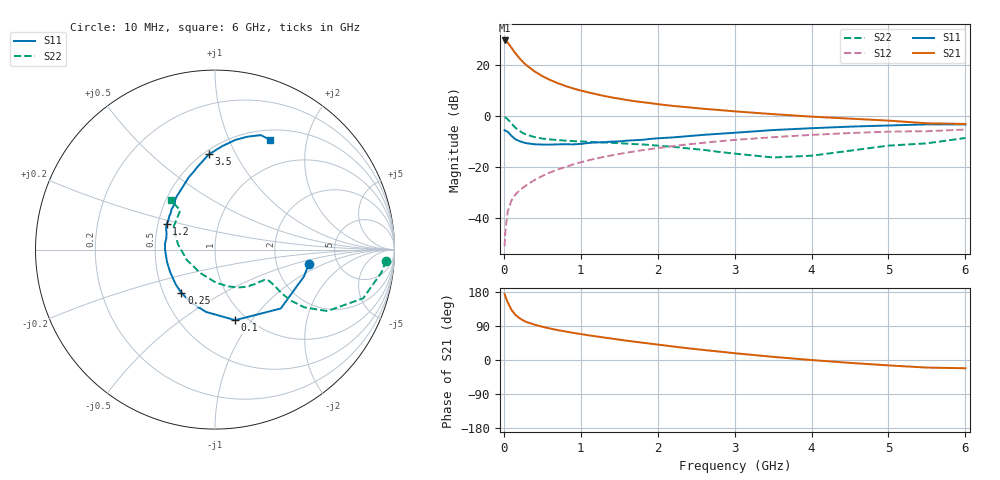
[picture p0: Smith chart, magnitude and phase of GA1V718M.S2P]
! Infineon Technologies  Discrete & RF Semiconductors
! BF775
! Si NPN RF Bipolar Junction Transistor in SOT23
! VCE = 1.75 V  IC = 18 mA
! Common Emitter S-Parameters:  May  1996
# GHz  S  MA  R  50
!  f  S11  S21  S12  S22
! GHz  MAG  ANG  MAG  ANG  MAG  ANG  MAG  ANG
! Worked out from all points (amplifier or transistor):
!   36 points, 10 MHz to 6 GHz, reference 50 ohm
!   highest |S21| = 29.7 dB at 10 MHz (marker M1)
!   |S21| within 3 dB of that: start of sweep to 102.4 MHz
!   unconditionally stable (mu >= 1): 350.1 MHz to 4.117 GHz; 5.266 GHz to end of sweep
!   at 250 MHz: K = 0.89, MSG = 24.6 dB, |S12| = -28.1 dB
!   at 1.4 GHz: K = 1.15, MAG = 9.1 dB, |S12| = -15.4 dB
!   at 6 GHz: K = 1.00, MAG = 0.8 dB, |S12| = -5.3 dB
!   S11 on the Smith chart (normalised r, x): 10 MHz: 3.07, -0.71; 100 MHz: 0.88, -0.83; 250 MHz: 0.62, -0.33; 1.2 GHz: 0.56, +0.17; 3.5 GHz: 0.53, +0.79; 6 GHz: 0.62, +1.43
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0.01  0.5292 -9.0  30.48 173.9  0.0028 85.6  0.9553 -3.7
0.02  0.5174 -16.9  30.07 167.9  0.0055 82.8  0.9362 -7.8
0.05  0.492 -41.8  27.62 152.1  0.0133 75.3  0.8689 -18.2
0.1  0.409 -74.0  21.83 132.3  0.0223 65.6  0.7133 -28.7
0.15  0.351 -98.1  17.1 119.1  0.0289 63.7  0.5924 -32.9
0.2  0.3239 -114.5  13.84 110.8  0.0342 63.5  0.5163 -33.8
0.25  0.3053 -127.7  11.45 104.6  0.0395 64.2  0.4635 -33.5
0.3  0.2924 -138.4  9.76 99.9  0.0447 65.4  0.4289 -32.8
0.4  0.2796 -153.3  7.529 93.3  0.0557 66.9  0.3872 -31.2
0.5  0.2761 -164.5  6.087 87.7  0.0667 67.9  0.3622 -30.4
0.6  0.2755 -173.8  5.125 83.1  0.078 68.2  0.3482 -30.0
0.7  0.2784 179.4  4.433 78.9  0.0894 68.2  0.3382 -30.2
0.8  0.2806 173.1  3.897 75.2  0.1006 67.6  0.3296 -30.8
0.9  0.2783 167.5  3.493 71.7  0.1126 67.0  0.323 -31.5
1.1  0.2965 156.8  2.911 65.3  0.1357 65.8  0.313 -34.3
1.2  0.3045 152.4  2.688 62.2  0.1468 64.8  0.307 -35.6
1.6  0.3293 137.4  2.067 50.9  0.1919 60.5  0.2875 -42.9
2.2  0.3815 120.2  1.582 35.7  0.2576 53.2  0.2495 -57.7
3.5  0.5317 93.7  1.092 8.3  0.3856 35.2  0.1541 -121.5
4.5  0.6208 79.6  0.891 -7.6  0.4645 21.2  0.2092 171.5
5.5  0.6871 68.2  0.722 -20.0  0.5044 6.7  0.2919 131.6
6  0.6845 63.3  0.701 -21.8  0.5442 2.6  0.3721 131.6
